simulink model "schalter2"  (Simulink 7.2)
settings: Solver=FixedStepDiscrete  StartTime=0.0  StopTime=100  FixedStep=0.0001  RelTol=1e-3
libraries: simulink x1

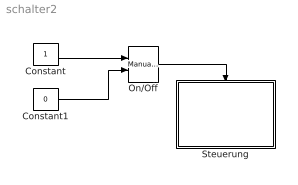
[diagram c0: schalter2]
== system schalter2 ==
  Constant : Constant  OutDataType=sfix(16)  OutScaling=2^0
  Constant1 : Constant  Value=0  OutDataType=sfix(16)  OutScaling=2^0
  On/Off : simulink/Signal Routing/Manual Switch  SystemSampleTime=-1  sw=1  action=0  varsize=off
  Steuerung : Stateflow chart  TreatAsAtomicUnit=on
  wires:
  Constant1/1 -> On/Off/2
  Constant/1 -> On/Off/1
  On/Off/1 -> Steuerung/Trigger

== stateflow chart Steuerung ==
  state Ein
  state Aus
  Ein -> Aus : schalten
  Aus -> Ein : schalten
  (default) -> Aus
